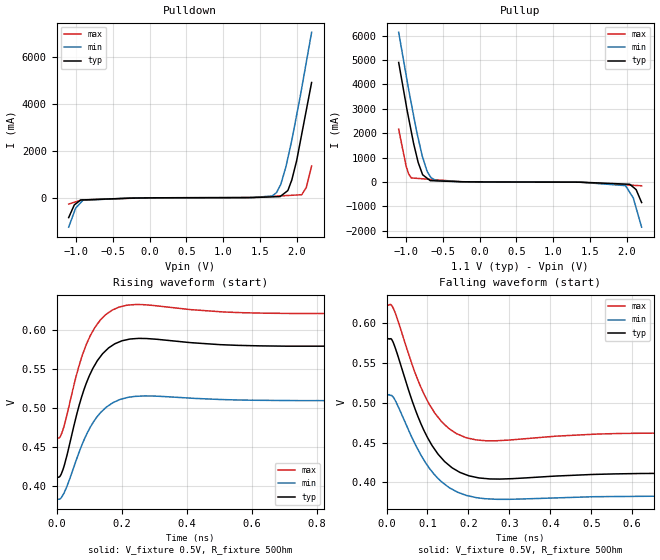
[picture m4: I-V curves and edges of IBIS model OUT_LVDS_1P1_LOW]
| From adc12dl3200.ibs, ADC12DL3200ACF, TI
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|   OUT_LVDS_1P1_LOW
[Model]   OUT_LVDS_1P1_LOW
Model_type   Output
Polarity   Non-Inverting
Vmeas = 0.5
Vref = 0.5
Cref = 2pF
Rref = 50
|   typ   min   max
C_comp   1.736E-12   1.689E-12   1.736E-12
[Voltage Range]   1.1   1.05   1.15
[Temperature Range]   90   150   -55
[Pullup Reference]   1.1   1.05   1.15
[Pulldown Reference]   0   -0   -0
[Power Clamp Reference]   1.1   1.05   1.15
[GND Clamp Reference]   0   0   0
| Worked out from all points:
|   slope of the pulldown table from 0 to 0.165 V, typ, clamps not added: 47 ohm
|   slope of the pullup table from 0 to 0.165 V, typ, clamps not added: 69.8 ohm
|   falling waveform, V_fixture 0.5V, R_fixture 50Ohm: 20-80 % time 77.2ps typ, 81.7ps min, 73.2ps max; typ from 0.579 V to 0.412 V
|   rising waveform, V_fixture 0.5V, R_fixture 50Ohm: 20-80 % time 70.4ps typ, 76.8ps min, 66.4ps max; typ from 0.412 V to 0.579 V
[Pulldown]
|   Voltage   I(typ)   I(min)   I(max)
-1.1V     -841.8mA   -1.249A    -267.7mA
-1.005V   -257.9mA   -436.8mA   -172.1mA
-905.6mV  -90.26mA   -105.5mA   -93.22mA
1.391V    9.928mA    9.569mA    15.26mA
1.723V    44.58mA    220.7mA    71.18mA
1.785V    81.18mA    602.7mA    81.46mA
1.875V    300.7mA    1.658A     96.67mA
1.931V    755.3mA    2.447A     106.1mA
1.997V    1.576A     3.516A     117.2mA
2.066V    2.713A     4.674A     132.1mA
2.129V    3.73A      5.771A     441.5mA
2.2V      4.899A     7.032A     1.354A
[Pullup]
|   Voltage   I(typ)   I(min)   I(max)
-1.1V     4.899A     6.134A     2.161A
-1.001V   3.211A     4.425A     685.7mA
-929.2mV  2.072A     3.227A     166.4mA
-835.3mV  802.5mA    1.798A     145mA
-776.2mV  310.2mA    1.031A     131.5mA
-717.1mV  162.6mA    466.3mA    118mA
-662.6mV  54.41mA    184.4mA    105.6mA
-254.8mV  11.04mA    10.42mA    12.52mA
1.979V    -85.45mA   -147.9mA   -117.1mA
2.087V    -213.4mA   -651.5mA   -135.5mA
2.126V    -311.4mA   -1.063A    -142.2mA
2.2V      -841.8mA   -1.851A    -154.9mA
[Ramp]
R_load = 50
|   typ   min   max
dV/dt_r   0.100407/7.03781e-11  0.0755354/7.67538e-11  0.0953078/6.63994e-11
dV/dt_f   0.100394/7.71168e-11  0.0755241/8.16821e-11  0.0952999/7.31505e-11
[Falling Waveform]
V_fixture = 0.5V
V_fixture_min = 0.45V
V_fixture_max = 0.55V
R_fixture = 50Ohm
C_fixture = 0F
|   Time   V(typ)   V(min)   V(max)
0s        578.9mV    509mV      620.9mV
10.29ps   579.9mV    509mV      622.6mV
16.81ps   574.6mV    506.6mV    617.6mV
76.75ps   482.5mV    441.3mV    528mV
103.8ps   452.8mV    418.4mV    498.3mV
126.1ps   435.3mV    404.9mV    481.5mV
170.7ps   415.2mV    388.6mV    461.2mV
252.5ps   404.4mV    379.4mV    452.2mV
734.2ps   411.6mV    383.2mV    462.1mV
5ns       411.6mV    383.2mV    462mV
[Rising Waveform]
V_fixture = 0.5V
V_fixture_min = 0.45V
V_fixture_max = 0.55V
R_fixture = 50Ohm
C_fixture = 0F
|   Time   V(typ)   V(min)   V(max)
0s        411.6mV    383.2mV    462mV
10ps      411.6mV    382.8mV    462mV
19.73ps   420.5mV    388.1mV    471.7mV
66.45ps   498.2mV    439.5mV    549.8mV
103.8ps   543.5mV    475.1mV    592.5mV
126.1ps   560.6mV    489.1mV    607.6mV
160.2ps   576.7mV    502.7mV    621.9mV
225.9ps   588.1mV    513.6mV    631.8mV
734.2ps   578.9mV    509.1mV    620.8mV
5ns       578.9mV    509.1mV    620.9mV
